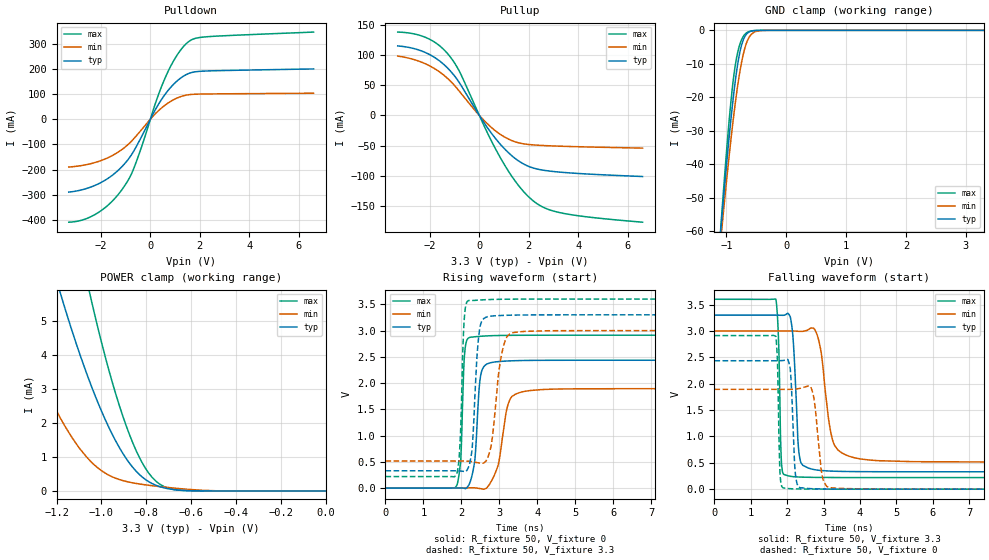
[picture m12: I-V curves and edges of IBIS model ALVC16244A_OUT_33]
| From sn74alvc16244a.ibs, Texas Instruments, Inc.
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[Model]   ALVC16244A_OUT_33
Model_type  3-state
Enable   Active-Low
Vref =   0
Rref =   500
Cref =   50p
Vmeas =   1.5
| variable   typ   min   max
C_comp   2.36pF   2.06pF   2.49pF
| C_pullup   3.37pF   2.73pF   4.38pF
| C_pulldown   4.25pF   2.14pF   6.78pF
| C_tri-state   2.36pF   2.06pF   2.49pF
[Temperature Range]   40   100   -40
| Ambient temperature   25   85   -40
[Voltage range]   3.3   3   3.6
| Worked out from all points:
|   slope of the pulldown table from 0 to 0.495 V, typ, clamps not added: 5.84 ohm
|   slope of the pullup table from 0 to 0.495 V, typ, clamps not added: 16.6 ohm
|   GND clamp passes 1 mA (typ) near -0.66 V on its own axis
|   POWER clamp passes 1 mA (typ) near -0.89 V on its own axis
|   rising waveform, R_fixture 50, V_fixture 0: 20-80 % time 129ps typ, 260ps min, 79.1ps max; typ from 0 V to 2.44 V
|   falling waveform, R_fixture 50, V_fixture 3.3: 20-80 % time 119ps typ, 267ps min, 64.7ps max; typ from 3.3 V to 0.33 V
|   rising waveform, R_fixture 50, V_fixture 3.3: 20-80 % time 133ps typ, 227ps min, 87.2ps max; typ from 0.33 V to 3.3 V
|   falling waveform, R_fixture 50, V_fixture 0: 20-80 % time 88ps typ, 158ps min, 52.4ps max; typ from 2.44 V to 0 V
[GND Clamp]
| ALVC16244A_OUT_33
|   Voltage   I(typ)   I(min)   I(max)
-3.3V     -647.6mA   -588.6mA   -724.5mA
-1.09V    -58.9mA    -61.92mA   -57.94mA
-1.07V    -54.69mA   -58.15mA   -53.03mA
-950mV    -31.09mA   -36.84mA   -26.11mA
-860mV    -16.35mA   -22.92mA   -11.42mA
-815mV    -10.55mA   -16.95mA   -6.862mA
-755mV    -4.988mA   -10.33mA   -3.168mA
-695mV    -1.948mA   -5.513mA   -1.265mA
-635mV    -657.5uA   -2.546mA   -444.5uA
-530mV    -83.99uA   -504.9uA   -65.23uA
-350mV    -2.358uA   -23.5uA    -2.845uA
3.3V      1.975nA    74.79nA    9.615nA
[POWER Clamp]
| ALVC16244A_OUT_33
|   Voltage   I(typ)   I(min)   I(max)
-3.3V     98.9mA     67.86mA    143.4mA
-1.43V    12.27mA    5.912mA    20.35mA
-1.405V   11.53mA    5.461mA    19.19mA
-1.18V    5.742mA    2.103mA    9.959mA
-1.065V   3.433mA    987.7uA    6.182mA
-1.045V   3.081mA    848uA      5.599mA
-950mV    1.639mA    409.1uA    3.155mA
-875mV    815.2uA    256.5uA    1.654mA
-820mV    418.5uA    193.5uA    847.4uA
-755mV    160.1uA    138.5uA    273.4uA
-650mV    20.91uA    67.11uA    18.91uA
-48.03fV  1.975nA    59.68nA    9.136nA
[Pulldown]
| ALVC16244A_OUT_33
|   Voltage   I(typ)   I(min)   I(max)
-3.3V     -289.4mA   -189.9mA   -408.8mA
-2.685V   -278.1mA   -182.3mA   -398.1mA
-2.08V    -255.5mA   -167.1mA   -368.8mA
-1.52V    -221.2mA   -143.2mA   -323.1mA
-1.03V    -175.5mA   -111.2mA   -262.7mA
-605mV    -114.8mA   -70.11mA   -178.6mA
240mV     44.44mA    25.45mA    73.3mA
610mV     100.6mA    56.89mA    166.8mA
1.075V    151.3mA    83.7mA     253.6mA
1.535V    180.8mA    96.88mA    306.9mA
2.285V    191.4mA    100.1mA    327.2mA
6.6V      199.5mA    103.1mA    345.7mA
[Pullup]
| ALVC16244A_OUT_33
|   Voltage   I(typ)   I(min)   I(max)
-3.3V     115.4mA    98.49mA    138.4mA
-2.1V     102.9mA    84.17mA    128.2mA
-1.625V   91.01mA    72.67mA    116.2mA
-1.215V   75.74mA    58.82mA    99.26mA
-775mV    52.22mA    38.43mA    70.63mA
80mV      -5.193mA   -3.635mA   -7.301mA
680mV     -39.7mA    -26.5mA    -57.58mA
1.47V     -72.16mA   -44.16mA   -110.2mA
2.215V    -87.78mA   -49.09mA   -143.1mA
2.72V     -91.81mA   -50.28mA   -155mA
3.43V     -94.82mA   -51.36mA   -162.9mA
6.6V      -101.5mA   -54.33mA   -177.4mA
[Ramp]
| ALVC16244A_OUT_33
| variable   typ   min   max
dV/dt_r   1.47/1.34E-10   1.15/2.79E-10   1.75/8.29E-11
dV/dt_f   1.80/1.25E-10   1.52/2.78E-10   2.03/6.87E-11
R_load = 50
[Rising Waveform]
| ALVC16244A_OUT_33
R_fixture =   50
C_fixture =   0
L_fixture =   0
V_fixture =   0
V_fixture_min = 0
V_fixture_max = 0
|   Time   V(typ)   V(min)   V(max)
0s        301.6pV    455.6pV    207.3pV
1.87ns    1.478mV    -63.79uV   39.96mV
1.985ns   3.055mV    398.7uV    547.2mV
2.11ns    -10.47mV   1.798mV    2.716V
2.355ns   524.9mV    4.087mV    2.882V
2.47ns    1.903V     -6.161mV   2.889V
2.955ns   2.408V     403.1mV    2.906V
3.31ns    2.424V     1.723V     2.909V
4.11ns    2.433V     1.876V     2.911V
50ns      2.435V     1.893V     2.912V
[Falling Waveform]
| ALVC16244A_OUT_33
R_fixture =   50
C_fixture =   0
L_fixture =   0
V_fixture =   3.3
V_fixture_min = 3
V_fixture_max = 3.6
|   Time   V(typ)   V(min)   V(max)
0s        3.3V       3V         3.6V
1.69ns    3.299V     3V         3.597V
1.765ns   3.298V     3V         2.743V
1.85ns    3.297V     3V         430.1mV
2.145ns   2.98V      2.998V     238.4mV
2.36ns    538.8mV    2.991V     229.2mV
2.975ns   351.5mV    2.358V     222.1mV
3.305ns   340.1mV    825.6mV    221.1mV
4.505ns   330.9mV    539.9mV    220.2mV
50ns      329.8mV    515mV      220.1mV
[Rising Waveform]
| ALVC16244A_OUT_33
R_fixture =   50
C_fixture =   0
L_fixture =   0
V_fixture =   3.3
V_fixture_min = 3
V_fixture_max = 3.6
|   Time   V(typ)   V(min)   V(max)
0s        329.8mV    515mV      220.1mV
1.88ns    328.9mV    515.7mV    280.1mV
1.97ns    325.8mV    515.7mV    928mV
2.075ns   315.6mV    514.9mV    3.197V
2.2ns     419.1mV    510.8mV    3.575V
2.48ns    3.014V     477.9mV    3.582V
2.785ns   3.276V     806.3mV    3.592V
3.125ns   3.289V     2.74V      3.597V
3.66ns    3.297V     2.985V     3.599V
50ns      3.3V       3V         3.6V
[Falling Waveform]
| ALVC16244A_OUT_33
R_fixture =   50
C_fixture =   0
L_fixture =   0
V_fixture =   0
V_fixture_min = 0
V_fixture_max = 0
|   Time   V(typ)   V(min)   V(max)
0s        2.435V     1.893V     2.912V
1.685ns   2.435V     1.893V     2.899V
1.73ns    2.435V     1.893V     2.447V
1.81ns    2.436V     1.892V     212.2mV
2.04ns    2.413V     1.892V     11.25mV
2.235ns   235.1mV    1.898V     5.181mV
2.565ns   13.21mV    1.953V     2.15mV
2.99ns    3.501mV    172.3mV    759.1uV
3.455ns   1.162mV    14.54mV    254.8uV
50ns      15.22nV    -7.871nV   -320.1pV
